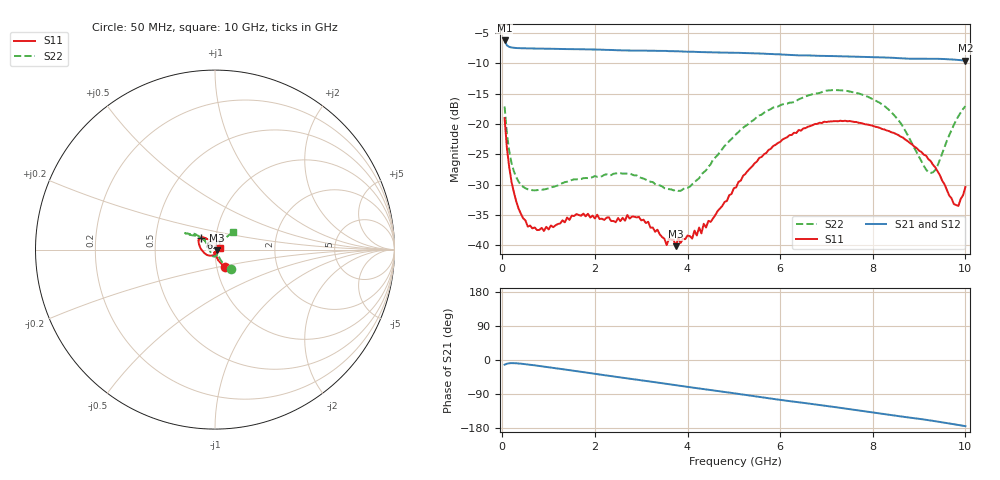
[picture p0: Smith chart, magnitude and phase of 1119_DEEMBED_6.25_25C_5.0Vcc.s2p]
!Hittite Microwave Corp.
!Digital Attenuator/PhaseShifter Rev 1.4.0
!Filename: C:\DATA\DATA\1119_DEEMBED_6.25_25C_5.0Vcc.s2p
!VNA ID: Agilent Technologies,N5224A,MY51441122,A.10.45.03
!Device type:
!2 Port Calibration.
!Temp(C): 25
!Lot Number:
!Serial Number:
!Operator:
!Misc:
!Attenuator:  6.250
# GHZ S DB R 50.0
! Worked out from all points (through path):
!   200 points, 50 MHz to 10 GHz, reference 50 ohm
!   highest |S21| = -6.21 dB at 50 MHz (marker M1); lowest = -9.5 dB at 10 GHz (marker M2)
!   group delay of S21, straight-line fit = 47.2 ps
!   lowest |S11| = -40.2 dB at 3.75 GHz (marker M3), VSWR 1.02, Z = 50.9 - j0.44 ohm
!   |S11| at or under -10 dB: start of sweep to end of sweep
!   |S22| runs from -31.0 to -14.4 dB; largest |S21 - S12| = 0.0011
!   S11 on the Smith chart (normalised r, x): 50 MHz: 1.09, -0.22; 6.9 GHz: 0.85, +0.11; 10 GHz: 1.06, +0.01
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0.05  -19.03 -61.7  -6.21 -12.3  -6.21 -12.3  -17.12 -50.9
0.1  -24.02 -72.8  -7.03 -9.8  -7.02 -9.8  -21.58 -60.4
0.2  -29.59 -79.3  -7.37 -8.2  -7.37 -8.2  -26.46 -61.8
0.35  -33.95 -80.4  -7.48 -9.1  -7.48 -9.1  -29.50 -57.6
0.55  -36.95 -84.0  -7.52 -11.8  -7.52 -11.8  -30.78 -56.2
0.9  -37.67 -90.3  -7.57 -17.4  -7.57 -17.4  -30.81 -60.8
1.75  -34.80 -100.5  -7.67 -32.0  -7.67 -32.0  -28.95 -79.0
2.95  -35.35 -79.5  -7.88 -52.5  -7.89 -52.5  -28.77 -116.8
3.4  -38.22 -63.7  -7.93 -60.3  -7.93 -60.4  -30.13 -134.2
3.75  -40.18 -26.2  -8.00 -66.5  -8.00 -66.6  -30.86 -153.1
3.8  -38.80 -23.8  -8.00 -67.4  -8.01 -67.5  -31.04 -157.6
4.3  -38.06 26.3  -8.13 -75.9  -8.14 -76.0  -28.30 162.6
5.05  -30.46 90.9  -8.25 -88.6  -8.27 -88.7  -21.68 138.0
5.85  -23.64 124.0  -8.46 -102.6  -8.48 -102.7  -17.29 141.7
6.7  -20.20 136.6  -8.71 -116.4  -8.72 -116.4  -15.08 149.4
6.9  -19.84 138.9  -8.75 -119.5  -8.77 -119.6  -14.74 151.1
7.7  -19.81 153.4  -8.89 -133.2  -8.90 -133.2  -14.97 151.4
8.35  -21.18 167.6  -9.05 -144.5  -9.06 -144.5  -17.67 144.3
9.25  -26.12 -138.3  -9.23 -159.7  -9.24 -159.7  -28.09 108.0
9.75  -33.22 -54.1  -9.37 -169.5  -9.39 -169.5  -20.17 47.1
9.85  -33.52 -23.4  -9.42 -171.5  -9.43 -171.5  -18.71 45.7
10  -30.41 13.3  -9.53 -174.6  -9.54 -174.6  -17.06 44.5
